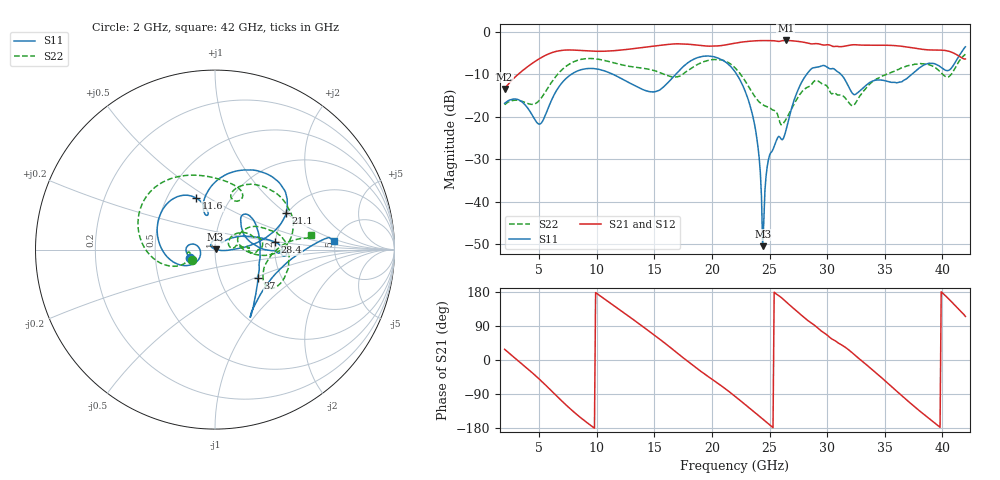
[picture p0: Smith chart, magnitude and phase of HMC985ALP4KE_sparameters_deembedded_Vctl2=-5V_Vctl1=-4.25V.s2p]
!s2p File: Measurements: S11, S21, S12, S22
# GHz S dB R 50.0
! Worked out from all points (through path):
!   401 points, 2 GHz to 42 GHz, reference 50 ohm
!   highest |S21| = -2.07 dB at 26.4 GHz (marker M1); lowest = -13.4 dB at 2 GHz (marker M2)
!   lowest |S11| = -50.4 dB at 24.4 GHz (marker M3), VSWR 1.01, Z = 50.3 + j0.064 ohm
!   |S11| at or under -10 dB: start of sweep to 7.806 GHz; 22.14 GHz to 28.23 GHz (6.089 GHz wide, 24.2 % of centre); 31.18 GHz to 37.36 GHz (6.178 GHz wide, 18 % of centre)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
!   |S22| runs from -21.9 to -5.3 dB; largest |S21 - S12| = 0.00084
!   S11 on the Smith chart (normalised r, x): 2 GHz: 0.76, -0.07; 11.6 GHz: 0.69, +0.44; 21.1 GHz: 1.97, +1.01; 28.4 GHz: 2.00, +0.19; 37 GHz: 1.52, -0.53; 42 GHz: 4.80, +0.81
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2  -16.84 -161.8  -13.44 28.2  -13.44 28.2  -17.16 -155.7
5  -21.73 -172.8  -6.38 -50.1  -6.38 -50.1  -16.19 -160.0
6.3  -14.83 -150.6  -4.76 -88.3  -4.77 -88.3  -11.05 -161.6
8.7  -8.90 150.2  -4.45 -154.6  -4.44 -154.6  -6.48 151.3
11.6  -10.28 110.2  -4.45 140.9  -4.45 141.0  -7.41 103.5
13.6  -13.11 101.1  -3.85 97.1  -3.85 97.1  -8.45 75.9
15.4  -13.80 105.7  -3.25 56.4  -3.25 56.4  -9.54 62.5
17.9  -7.33 80.0  -2.95 -3.6  -2.95 -3.6  -9.14 72.3
21.1  -7.00 27.4  -3.14 -74.5  -3.14 -74.5  -6.88 16.1
22  -9.42 16.7  -2.71 -95.7  -2.71 -95.7  -8.49 0.6
23.6  -20.53 -0.3  -2.18 -135.5  -2.18 -135.4  -14.75 -3.8
24  -27.24 -7.2  -2.11 -145.5  -2.11 -145.5  -16.22 1.8
24.4  -50.43 12.2  -2.09 -155.6  -2.09 -155.6  -17.18 7.6
25  -29.02 133.2  -2.12 -170.9  -2.11 -170.8  -17.86 11.0
26.4  -23.45 43.1  -2.06 154.4  -2.06 154.5  -20.73 33.0
28.4  -9.41 7.1  -2.74 102.5  -2.74 102.5  -12.93 18.3
28.7  -8.60 2.0  -2.88 96.3  -2.88 96.3  -12.22 16.6
32.5  -14.66 33.6  -3.08 10.5  -3.08 10.5  -16.64 29.0
35.4  -11.77 18.9  -3.21 -65.0  -3.20 -64.9  -9.79 19.4
37  -10.83 -33.6  -3.63 -108.0  -3.63 -108.0  -8.02 5.0
39.8  -8.20 -56.7  -4.33 -177.5  -4.33 -177.5  -9.39 -34.8
42  -3.56 4.1  -6.41 114.9  -6.42 115.0  -5.30 8.8
